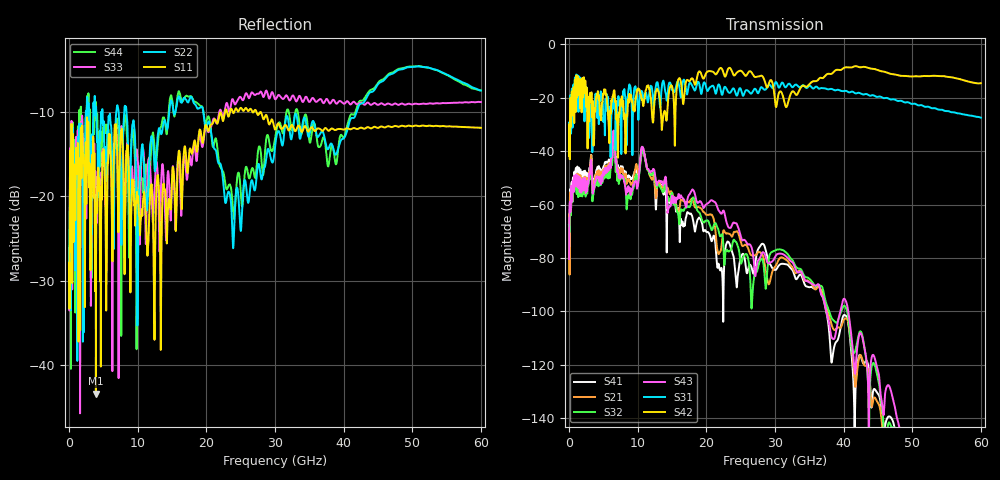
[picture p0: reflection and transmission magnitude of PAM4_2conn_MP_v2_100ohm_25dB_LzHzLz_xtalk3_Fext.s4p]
! Info: Touchstone file created by Circ.  Input file=FAB50GbE_2conn_Midplane_Examax_Topo2_v2_100ohm_25dB_LzHzLz.circ
# Hz S RI R 50
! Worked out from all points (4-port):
!   6000 points, 10 MHz to 60 GHz, reference 50 ohm
!   strongest paths, dB at 10 MHz, 15.01 GHz, 30.01 GHz, 45.01 GHz, 60 GHz:
!     S42: -41.8, -15.8, -21.2, -9.7, -14.6
!     S31: -41.2, -17.2, -14.4, -19.7, -27.5
!     S43: -80.4, -56.7, -79.6, -122.2, -175.6
!     S32: -67.5, -55.7, -77.2, -125.2, -184.7
!     S21: -63.8, -55.6, -83.3, -134.3, -184.4
!     S41: -66.9, -58.2, -84.5, -130.9, -187.1
!   lowest |S11| = -43.4 dB at 3.91 GHz (marker M1), VSWR 1.01, Z = 49.4 + j0.17 ohm
!   |S11| at or under -10 dB: start of sweep to 22.02 GHz; 22.06 GHz to 22.7 GHz (644.1 MHz wide, 2.88 % of centre); 27.96 GHz to end of sweep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
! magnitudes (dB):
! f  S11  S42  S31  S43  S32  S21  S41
! 10 MHz  -30.0  -41.8  -41.2  -80.4  -67.5  -63.8  -66.9
! 800 MHz  -16.6  -17.4  -15.3  -49.1  -54.2  -50.7  -47.9
! 3.91 GHz  -43.4  -20.6  -20.1  -50.9  -51.5  -48.8  -48.3
! 10.76 GHz  -20.8  -22.5  -19.6  -38.7  -39.8  -39.7  -38.6
! 21.77 GHz  -10.9  -9.8  -15.1  -62.1  -69.6  -78.5  -82.2
! 27.16 GHz  -9.7  -12.3  -16.7  -86.6  -85.2  -79.0  -81.0
! 60 GHz  -11.8  -14.6  -27.5  -175.6  -184.7  -184.4  -187.1
